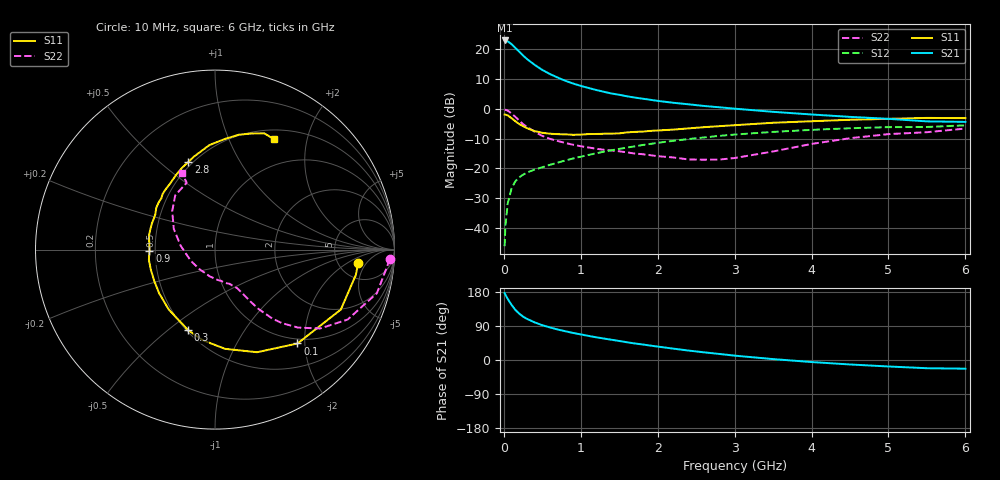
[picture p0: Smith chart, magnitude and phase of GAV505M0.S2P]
! Infineon Technologies  Discrete & RF Semiconductors
! BF775
! Si NPN RF Bipolar Junction Transistor in SOT23
! VCE = 0.5 V  IC = 5 mA
! Common Emitter S-Parameters:  May  1996
# GHz  S  MA  R  50
!  f  S11  S21  S12  S22
! GHz  MAG  ANG  MAG  ANG  MAG  ANG  MAG  ANG
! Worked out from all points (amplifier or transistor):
!   36 points, 10 MHz to 6 GHz, reference 50 ohm
!   highest |S21| = 23.0 dB at 10 MHz (marker M1)
!   |S21| within 3 dB of that: start of sweep to 169.2 MHz
!   unconditionally stable (mu >= 1): 626.2 MHz to end of sweep
!   at 250 MHz: K = 0.54, MSG = 20.1 dB, |S12| = -22.2 dB
!   at 1.4 GHz: K = 1.24, MAG = 6.6 dB, |S12| = -14.0 dB
!   at 6 GHz: K = 1.09, MAG = -1.2 dB, |S12| = -5.6 dB
!   S11 on the Smith chart (normalised r, x): 10 MHz: 7.74, -3.21; 100 MHz: 0.91, -1.85; 300 MHz: 0.51, -0.59; 900 MHz: 0.46, -0.01; 2.8 GHz: 0.47, +0.63; 6 GHz: 0.62, +1.48
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0.01  0.8018 -5.3  14.12 176.4  0.0049 86.4  0.9746 -3.1
0.02  0.7973 -10.2  13.83 172.3  0.0106 84.5  0.9615 -6.1
0.05  0.7765 -25.5  13.64 161.5  0.0255 76.8  0.934 -15.1
0.1  0.6963 -48.7  12.25 145.5  0.0457 65.7  0.8355 -27.8
0.15  0.618 -67.7  10.56 132.2  0.0607 57.9  0.7322 -36.9
0.2  0.5558 -84.2  9.149 122.3  0.0705 53.1  0.6346 -43.2
0.25  0.5097 -97.7  7.882 114.5  0.0779 50.1  0.5537 -47.7
0.3  0.4725 -108.6  6.889 108.6  0.0847 48.5  0.4987 -50.3
0.4  0.422 -127.6  5.494 99.3  0.0952 47.0  0.4116 -53.7
0.5  0.395 -141.9  4.505 91.8  0.1041 47.4  0.35 -55.7
0.6  0.3813 -152.4  3.84 85.9  0.1144 48.0  0.3127 -56.9
0.7  0.3747 -162.7  3.354 80.5  0.1245 48.2  0.2877 -57.9
0.9  0.3653 -178.6  2.663 71.4  0.1462 49.0  0.2488 -60.1
1.1  0.3761 167.9  2.243 63.6  0.1674 49.2  0.2239 -63.9
1.3  0.3807 157.5  1.935 56.7  0.19 48.5  0.2048 -67.8
1.6  0.4014 144.6  1.624 46.8  0.223 46.6  0.1854 -76.0
2.2  0.4469 123.5  1.266 30.1  0.2892 40.9  0.1522 -101.2
2.8  0.5107 106.9  1.062 16.0  0.3509 33.6  0.1401 -142.2
3.5  0.583 93.1  0.89 2.4  0.4093 24.0  0.1919 173.9
4.5  0.6542 78.2  0.732 -11.8  0.4714 10.8  0.3206 138.0
5.5  0.7037 67.0  0.615 -21.7  0.4951 -2.0  0.4045 112.9
6  0.6968 62.1  0.603 -22.9  0.5274 -5.6  0.4656 113.5
